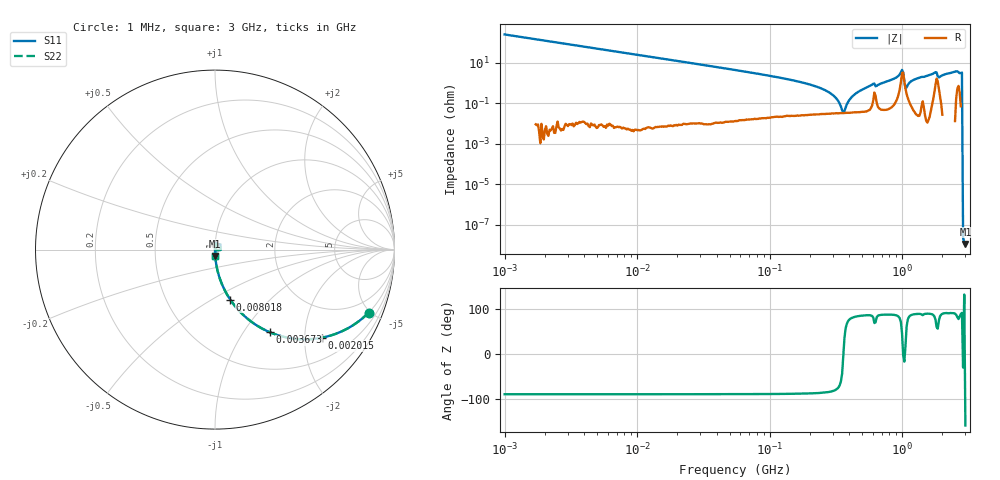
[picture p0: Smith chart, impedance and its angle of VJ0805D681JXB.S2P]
! VJ0805D681JXB
! DATE
! CORRECTED  DATA
# Hz  S  MA  R  50
!Freq	S11M	S11A	S21M	S21A	S12M	S12A	S22M	S22A
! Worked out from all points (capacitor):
!   401 points, 1 MHz to 3 GHz, reference 50 ohm
!   read as one part in series: C = 652 pF near 1.041 MHz
!   lowest |Z| = 11.6 nohm at 3 GHz (marker M1)
!   series resonance near 360.4 MHz, so ESL is about 300 pH
!   S11 on the Smith chart (normalised r, x): 1 MHz: 1.00, -4.88; 2.015 MHz: 1.00, -2.42; 3.673 MHz: 1.00, -1.33; 8.018 MHz: 1.00, -0.61; 3 GHz: 1.00, -0.07
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1000000  0.9253 -22.3  0.3793 67.7  0.3793 67.7  0.9253 -22.3
2014875  0.771 -39.6  0.6368 50.4  0.6368 50.4  0.771 -39.6
3673095  0.5532 -56.4  0.833 33.6  0.833 33.6  0.5532 -56.4
3823119  0.5378 -57.5  0.843 32.5  0.843 32.5  0.5378 -57.5
8017732  0.2909 -73.1  0.9567 16.9  0.9567 16.9  0.2909 -73.1
1.461624e7  0.1643 -80.5  0.9863 9.5  0.9863 9.5  0.1643 -80.5
5.587962e7  0.04249 -87.4  0.999 2.4  0.999 2.4  0.04249 -87.4
2.094008e8  0.007692 -87.5  0.9997 0.4  0.9997 0.4  0.007692 -87.5
2.942768e8  0.002777 -83.3  0.9997 0.2  0.9997 0.2  0.002777 -83.3
3.594878e8  0.0003297 -6.1  0.9997 0.0  0.9997 0.0  0.0003297 -6.1
4.135554e8  0.00192 79.6  0.9997 -0.1  0.9997 -0.1  0.00192 79.6
4.66327e8  0.003638 84.1  0.9996 -0.2  0.9996 -0.2  0.003638 84.1
5.929311e8  0.008152 84.2  0.9992 -0.5  0.9992 -0.5  0.008152 84.2
8.005644e8  0.01306 86.9  0.9994 -0.7  0.9994 -0.7  0.01306 86.9
9.779672e8  0.03271 69.2  0.9889 -1.8  0.9889 -1.8  0.03271 69.2
1.080907e9  0.006005 61.6  0.9972 -0.3  0.9972 -0.3  0.006005 61.6
1.10276e9  0.007959 76.5  0.9982 -0.4  0.9982 -0.4  0.007959 76.5
1.243477e9  0.01493 87.8  0.9995 -0.9  0.9995 -0.9  0.01493 87.8
1.747494e9  0.03109 82.3  0.9963 -1.8  0.9963 -1.8  0.03109 82.3
1.931433e9  0.02036 82.8  0.9977 -1.2  0.9977 -1.2  0.02036 82.8
2.505452e9  0.03554 87.8  0.9992 -2.0  0.9992 -2.0  0.03554 87.8
3e9  0.03614 -88.4  1.002 -2.1  1.002 -2.1  0.03614 -88.4
